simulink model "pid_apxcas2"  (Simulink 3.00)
settings: Solver=ode45  SolverMode=SingleTasking  StartTime=0.0  StopTime=200  FixedStep=st_size  MaxStep=st_size  RelTol=1e-5  AbsTol=1e-6
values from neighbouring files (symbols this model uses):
  Disturb = Setpoint    [mimo_MSF1DF_sim.m]    (also in mimo_MSF2DF_sim.m)
  Satlb = temp1    [cback.m]    (also in imcmenu.m = str2num(satlbs))
  Satub = temp1    [cback.m]    (also in imcmenu.m = str2num(satubs))
  Setpoint = zeros(1,n)    [mimo_MSF1DF_sim.m]    (also in mimo_MSF2DF_sim.m)
undefined symbols (not defined in the file or in its folder): a1, a2, b1, b2, keps, Pre_fil_den, Pre_fil_num, XdenMs, XdenPs, Xmdeadx, XnumMs, XnumPs, Xpdeadx

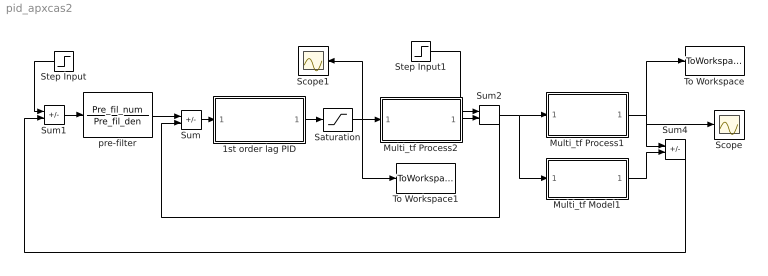
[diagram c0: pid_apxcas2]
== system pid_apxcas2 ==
  1st order lag PID : Subsystem
  Multi_tf Model1 : Subsystem
  Multi_tf Process1 : Subsystem
  Multi_tf Process2 : Subsystem
  Saturation : Saturate  UpperLimit=Satub  LowerLimit=Satlb
  Scope : Scope
  Scope1 : Scope
  Step Input : Step  Orientation=left  Time=0  Before=0  After=Setpoint  SampleTime=0
  Step Input1 : Step  Time=0  Before=0  After=Disturb  SampleTime=0
  Sum : Sum  Inputs=+-  SaturateOnIntegerOverflow=on
  Sum1 : Sum  Inputs=+-  SaturateOnIntegerOverflow=on
  Sum2 : Sum  Inputs=++  SaturateOnIntegerOverflow=on
  Sum4 : Sum  Inputs=+-  SaturateOnIntegerOverflow=on
  To Workspace : ToWorkspace  VariableName=simout  SampleTime=-1  SaveFormat=Matrix
  To Workspace1 : ToWorkspace  VariableName=effort  SampleTime=-1  SaveFormat=Matrix
  pre-filter : TransferFcn  Numerator=Pre_fil_num  Denominator=Pre_fil_den
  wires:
  pre-filter/1 -> Sum/1
  Sum/1 -> 1st order lag PID/1(In1)
  Multi_tf Process2/1(Out1) -> Sum2/2
  Step Input1/1 -> Sum2/1
  1st order lag PID/1(Out1) -> Saturation/1
  Saturation/1 -> To Workspace1/1, Multi_tf Process2/1(In1), Scope1/1
  Sum2/1 -> Sum/2, Multi_tf Process1/1(In1), Multi_tf Model1/1(In1)
  Multi_tf Model1/1(Out1) -> Sum4/2
  Multi_tf Process1/1(Out1) -> Sum4/1, To Workspace/1, Scope/1
  Sum1/1 -> pre-filter/1
  Step Input/1 -> Sum1/1
  Sum4/1 -> Sum1/2

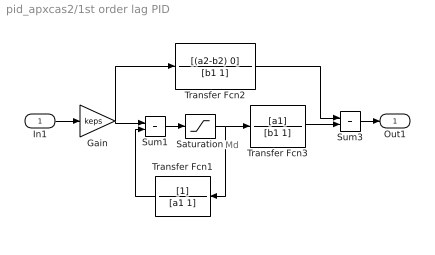
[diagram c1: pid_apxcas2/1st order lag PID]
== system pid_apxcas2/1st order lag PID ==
  note: Md
  In1 : Inport  Port=1  PortWidth=-1  SampleTime=-1  DataType=auto
  Gain : Gain  Gain=keps  SaturateOnIntegerOverflow=on
  Saturation : Saturate  UpperLimit=Satub  LowerLimit=Satlb
  Sum1 : Sum  Inputs=++  SaturateOnIntegerOverflow=on
  Sum3 : Sum  Inputs=++  SaturateOnIntegerOverflow=on
  Transfer Fcn1 : TransferFcn  Orientation=left  Numerator=[1]  Denominator=[a1 1]
  Transfer Fcn2 : TransferFcn  Numerator=[(a2-b2) 0]  Denominator=[b1 1]
  Transfer Fcn3 : TransferFcn  Numerator=[a1]  Denominator=[b1 1]
  Out1 : Outport  Port=1  InitialOutput=0
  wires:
  Gain/1 -> Transfer Fcn2/1, Sum1/1
  Transfer Fcn1/1 -> Sum1/2
  Saturation/1 -> Transfer Fcn1/1, Transfer Fcn3/1
  Sum1/1 -> Saturation/1
  Transfer Fcn3/1 -> Sum3/2
  In1/1 -> Gain/1
  Sum3/1 -> Out1/1
  Transfer Fcn2/1 -> Sum3/1

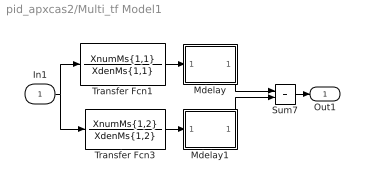
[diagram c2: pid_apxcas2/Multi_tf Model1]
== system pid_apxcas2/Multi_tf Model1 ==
  In1 : Inport  Port=1  PortWidth=-1  SampleTime=-1  DataType=auto
  Mdelay : Subsystem
  Mdelay1 : Subsystem
  Sum7 : Sum  Inputs=++  SaturateOnIntegerOverflow=on
  Transfer Fcn1 : TransferFcn  Numerator=XnumMs{1,1}  Denominator=XdenMs{1,1}
  Transfer Fcn3 : TransferFcn  Numerator=XnumMs{1,2}  Denominator=XdenMs{1,2}
  Out1 : Outport  Port=1  InitialOutput=0
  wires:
  Transfer Fcn1/1 -> Mdelay/1(In1)
  Transfer Fcn3/1 -> Mdelay1/1(In1)
  In1/1 -> Transfer Fcn1/1, Transfer Fcn3/1
  Sum7/1 -> Out1/1
  Mdelay/1(Out1) -> Sum7/1
  Mdelay1/1(Out1) -> Sum7/2

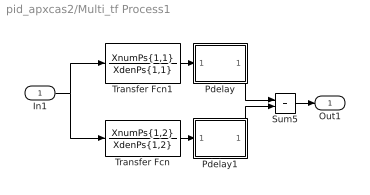
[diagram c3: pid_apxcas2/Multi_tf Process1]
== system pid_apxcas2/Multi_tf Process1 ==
  In1 : Inport  Port=1  PortWidth=-1  SampleTime=-1  DataType=auto
  Pdelay : Subsystem
  Pdelay1 : Subsystem
  Sum5 : Sum  Inputs=++  SaturateOnIntegerOverflow=on
  Transfer Fcn : TransferFcn  Numerator=XnumPs{1,2}  Denominator=XdenPs{1,2}
  Transfer Fcn1 : TransferFcn  Numerator=XnumPs{1,1}  Denominator=XdenPs{1,1}
  Out1 : Outport  Port=1  InitialOutput=0
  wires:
  Transfer Fcn1/1 -> Pdelay/1(In1)
  Transfer Fcn/1 -> Pdelay1/1(In1)
  Pdelay/1(Out1) -> Sum5/1
  In1/1 -> Transfer Fcn1/1, Transfer Fcn/1
  Sum5/1 -> Out1/1
  Pdelay1/1(Out1) -> Sum5/2

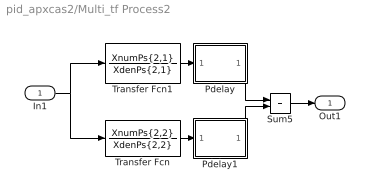
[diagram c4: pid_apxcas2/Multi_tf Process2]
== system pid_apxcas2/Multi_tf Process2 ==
  In1 : Inport  Port=1  PortWidth=-1  SampleTime=-1  DataType=auto
  Pdelay : Subsystem
  Pdelay1 : Subsystem
  Sum5 : Sum  Inputs=++  SaturateOnIntegerOverflow=on
  Transfer Fcn : TransferFcn  Numerator=XnumPs{2,2}  Denominator=XdenPs{2,2}
  Transfer Fcn1 : TransferFcn  Numerator=XnumPs{2,1}  Denominator=XdenPs{2,1}
  Out1 : Outport  Port=1  InitialOutput=0
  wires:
  Transfer Fcn1/1 -> Pdelay/1(In1)
  Transfer Fcn/1 -> Pdelay1/1(In1)
  Pdelay/1(Out1) -> Sum5/1
  Pdelay1/1(Out1) -> Sum5/2
  In1/1 -> Transfer Fcn1/1, Transfer Fcn/1
  Sum5/1 -> Out1/1

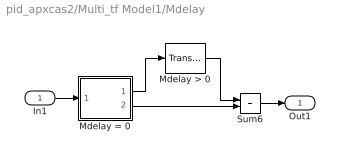
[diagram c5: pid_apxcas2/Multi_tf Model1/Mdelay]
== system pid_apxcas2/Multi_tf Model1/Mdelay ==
  In1 : Inport  Port=1  PortWidth=-1  SampleTime=-1  DataType=auto
  Mdelay > 0 : TransportDelay  DelayTime=Xmdeadx{1,1}  InitialInput=0  BufferSize=1024
  Mdelay = 0 : Subsystem  Description=pass input signal through out1 if condition is true.
  Sum6 : Sum  Inputs=++  SaturateOnIntegerOverflow=on
  Out1 : Outport  Port=1
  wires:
  Mdelay = 0/1(Out2) -> Mdelay > 0/1
  Mdelay > 0/1 -> Sum6/1
  Mdelay = 0/2(Out1) -> Sum6/2
  In1/1 -> Mdelay = 0/1(In)
  Sum6/1 -> Out1/1

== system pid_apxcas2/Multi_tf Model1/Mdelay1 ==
  In1 : Inport  Port=1  PortWidth=-1  SampleTime=-1  DataType=auto
  Mdelay > 0 : TransportDelay  DelayTime=Xmdeadx{1,2}  InitialInput=0  BufferSize=1024
  Mdelay = 0 : Subsystem  Description=pass input signal through out1 if condition is true.
  Sum6 : Sum  Inputs=++  SaturateOnIntegerOverflow=on
  Out1 : Outport  Port=1
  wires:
  Mdelay = 0/1(Out2) -> Mdelay > 0/1
  Mdelay > 0/1 -> Sum6/1
  Mdelay = 0/2(Out1) -> Sum6/2
  In1/1 -> Mdelay = 0/1(In)
  Sum6/1 -> Out1/1

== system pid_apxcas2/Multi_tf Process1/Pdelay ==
  In1 : Inport  Port=1  PortWidth=-1  SampleTime=-1  DataType=auto
  Mdelay > 0 : TransportDelay  DelayTime=Xpdeadx{1,1}  InitialInput=0  BufferSize=1024
  Mdelay = 0 : Subsystem  Description=pass input signal through out1 if condition is true.
  Sum6 : Sum  Inputs=++  SaturateOnIntegerOverflow=on
  Out1 : Outport  Port=1
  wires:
  Mdelay = 0/1(Out2) -> Mdelay > 0/1
  Mdelay > 0/1 -> Sum6/1
  Mdelay = 0/2(Out1) -> Sum6/2
  In1/1 -> Mdelay = 0/1(In)
  Sum6/1 -> Out1/1

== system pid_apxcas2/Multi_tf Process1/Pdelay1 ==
  In1 : Inport  Port=1  PortWidth=-1  SampleTime=-1  DataType=auto
  Mdelay > 0 : TransportDelay  DelayTime=Xpdeadx{1,2}  InitialInput=0  BufferSize=1024
  Mdelay = 0 : Subsystem  Description=pass input signal through out1 if condition is true.
  Sum6 : Sum  Inputs=++  SaturateOnIntegerOverflow=on
  Out1 : Outport  Port=1
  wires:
  Mdelay = 0/1(Out2) -> Mdelay > 0/1
  Mdelay > 0/1 -> Sum6/1
  Mdelay = 0/2(Out1) -> Sum6/2
  In1/1 -> Mdelay = 0/1(In)
  Sum6/1 -> Out1/1

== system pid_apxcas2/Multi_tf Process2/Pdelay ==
  In1 : Inport  Port=1  PortWidth=-1  SampleTime=-1  DataType=auto
  Mdelay > 0 : TransportDelay  DelayTime=Xpdeadx{2,1}  InitialInput=0  BufferSize=1024
  Mdelay = 0 : Subsystem  Description=pass input signal through out1 if condition is true.
  Sum6 : Sum  Inputs=++  SaturateOnIntegerOverflow=on
  Out1 : Outport  Port=1
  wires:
  Mdelay = 0/1(Out2) -> Mdelay > 0/1
  Mdelay > 0/1 -> Sum6/1
  Mdelay = 0/2(Out1) -> Sum6/2
  In1/1 -> Mdelay = 0/1(In)
  Sum6/1 -> Out1/1

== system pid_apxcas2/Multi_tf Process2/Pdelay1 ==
  In1 : Inport  Port=1  PortWidth=-1  SampleTime=-1  DataType=auto
  Mdelay > 0 : TransportDelay  DelayTime=Xpdeadx{2,2}  InitialInput=0  BufferSize=1024
  Mdelay = 0 : Subsystem  Description=pass input signal through out1 if condition is true.
  Sum6 : Sum  Inputs=++  SaturateOnIntegerOverflow=on
  Out1 : Outport  Port=1
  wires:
  Mdelay = 0/1(Out2) -> Mdelay > 0/1
  Mdelay > 0/1 -> Sum6/1
  Mdelay = 0/2(Out1) -> Sum6/2
  In1/1 -> Mdelay = 0/1(In)
  Sum6/1 -> Out1/1

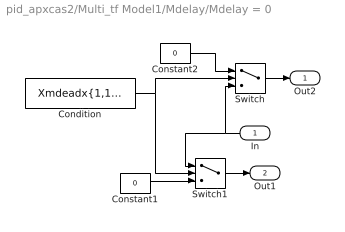
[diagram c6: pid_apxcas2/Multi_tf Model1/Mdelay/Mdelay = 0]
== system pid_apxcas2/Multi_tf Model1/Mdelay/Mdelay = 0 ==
  In : Inport  Orientation=left  Port=1  PortWidth=-1  SampleTime=-1  DataType=auto
  Condition : Constant  Value=Xmdeadx{1,1}<=3*eps
  Constant1 : Constant  Value=0
  Constant2 : Constant  Value=0
  Switch : Switch  Threshold=1
  Switch1 : Switch  Threshold=1
  Out2 : Outport  Port=1  InitialOutput=0
  Out1 : Outport  Port=2  InitialOutput=0
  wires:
  In/1 -> Switch/3, Switch1/1
  Condition/1 -> Switch1/2, Switch/2
  Constant1/1 -> Switch1/3
  Constant2/1 -> Switch/1
  Switch/1 -> Out2/1
  Switch1/1 -> Out1/1

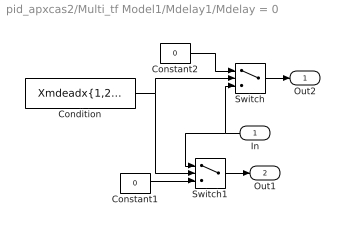
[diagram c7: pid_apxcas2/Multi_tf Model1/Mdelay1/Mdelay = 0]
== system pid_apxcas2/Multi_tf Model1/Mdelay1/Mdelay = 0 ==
  In : Inport  Orientation=left  Port=1  PortWidth=-1  SampleTime=-1  DataType=auto
  Condition : Constant  Value=Xmdeadx{1,2}<=3*eps
  Constant1 : Constant  Value=0
  Constant2 : Constant  Value=0
  Switch : Switch  Threshold=1
  Switch1 : Switch  Threshold=1
  Out2 : Outport  Port=1  InitialOutput=0
  Out1 : Outport  Port=2  InitialOutput=0
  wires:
  In/1 -> Switch/3, Switch1/1
  Condition/1 -> Switch1/2, Switch/2
  Constant1/1 -> Switch1/3
  Constant2/1 -> Switch/1
  Switch/1 -> Out2/1
  Switch1/1 -> Out1/1

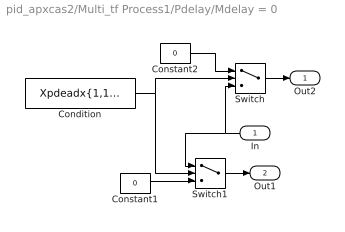
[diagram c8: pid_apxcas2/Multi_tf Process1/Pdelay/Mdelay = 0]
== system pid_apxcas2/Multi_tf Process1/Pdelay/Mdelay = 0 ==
  In : Inport  Orientation=left  Port=1  PortWidth=-1  SampleTime=-1  DataType=auto
  Condition : Constant  Value=Xpdeadx{1,1}<=3*eps
  Constant1 : Constant  Value=0
  Constant2 : Constant  Value=0
  Switch : Switch  Threshold=1
  Switch1 : Switch  Threshold=1
  Out2 : Outport  Port=1  InitialOutput=0
  Out1 : Outport  Port=2  InitialOutput=0
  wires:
  In/1 -> Switch/3, Switch1/1
  Condition/1 -> Switch1/2, Switch/2
  Constant1/1 -> Switch1/3
  Constant2/1 -> Switch/1
  Switch/1 -> Out2/1
  Switch1/1 -> Out1/1

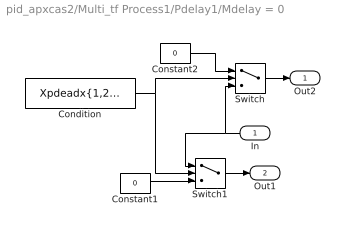
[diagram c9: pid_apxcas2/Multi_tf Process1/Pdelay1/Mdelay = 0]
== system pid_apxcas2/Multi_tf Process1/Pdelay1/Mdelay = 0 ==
  In : Inport  Orientation=left  Port=1  PortWidth=-1  SampleTime=-1  DataType=auto
  Condition : Constant  Value=Xpdeadx{1,2}<=3*eps
  Constant1 : Constant  Value=0
  Constant2 : Constant  Value=0
  Switch : Switch  Threshold=1
  Switch1 : Switch  Threshold=1
  Out2 : Outport  Port=1  InitialOutput=0
  Out1 : Outport  Port=2  InitialOutput=0
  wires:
  In/1 -> Switch/3, Switch1/1
  Condition/1 -> Switch1/2, Switch/2
  Constant1/1 -> Switch1/3
  Constant2/1 -> Switch/1
  Switch/1 -> Out2/1
  Switch1/1 -> Out1/1

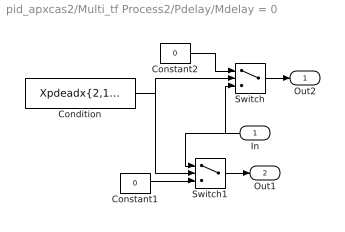
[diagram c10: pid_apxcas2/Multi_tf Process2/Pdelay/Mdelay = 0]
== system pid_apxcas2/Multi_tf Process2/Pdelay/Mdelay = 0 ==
  In : Inport  Orientation=left  Port=1  PortWidth=-1  SampleTime=-1  DataType=auto
  Condition : Constant  Value=Xpdeadx{2,1}<=3*eps
  Constant1 : Constant  Value=0
  Constant2 : Constant  Value=0
  Switch : Switch  Threshold=1
  Switch1 : Switch  Threshold=1
  Out2 : Outport  Port=1  InitialOutput=0
  Out1 : Outport  Port=2  InitialOutput=0
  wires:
  In/1 -> Switch/3, Switch1/1
  Condition/1 -> Switch1/2, Switch/2
  Constant1/1 -> Switch1/3
  Constant2/1 -> Switch/1
  Switch/1 -> Out2/1
  Switch1/1 -> Out1/1

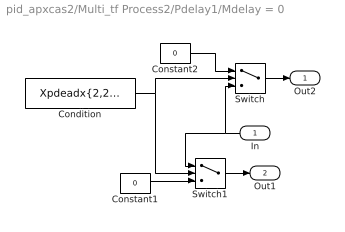
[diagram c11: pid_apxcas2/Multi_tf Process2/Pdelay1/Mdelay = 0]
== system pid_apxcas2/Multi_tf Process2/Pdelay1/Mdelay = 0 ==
  In : Inport  Orientation=left  Port=1  PortWidth=-1  SampleTime=-1  DataType=auto
  Condition : Constant  Value=Xpdeadx{2,2}<=3*eps
  Constant1 : Constant  Value=0
  Constant2 : Constant  Value=0
  Switch : Switch  Threshold=1
  Switch1 : Switch  Threshold=1
  Out2 : Outport  Port=1  InitialOutput=0
  Out1 : Outport  Port=2  InitialOutput=0
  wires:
  In/1 -> Switch/3, Switch1/1
  Condition/1 -> Switch1/2, Switch/2
  Constant1/1 -> Switch1/3
  Constant2/1 -> Switch/1
  Switch/1 -> Out2/1
  Switch1/1 -> Out1/1
